FUNCTION_BLOCK FB_DO_IED_LD1_MMXU1_TotW EXTENDS FB_AcsiCommonDataClass
VAR_INPUT
	mag: FB_AcsiDATypeAnalogueValue := (fc:=ACSI_FC_MX, TrgOp:=ACSI_TrgOp_dchg OR ACSI_TrgOp_dupd, bLinkResult:=THIS^.AddDataToContainer(ipData:=mag));
	q: FB_AcsiDATypeQuality := (fc:=ACSI_FC_MX, TrgOp:=ACSI_TrgOp_qchg, bLinkResult:=THIS^.AddDataToContainer(ipData:=q));
	t: FB_AcsiDATypeTimeStamp := (fc:=ACSI_FC_MX, bLinkResult:=THIS^.AddDataToContainer(ipData:=t));
	units: FB_AcsiDATypeUnit := (fc:=ACSI_FC_CF, TrgOp:=ACSI_TrgOp_dchg, SIUnit:=(eValue:=E_AcsiSIUnit.Volt), multiplier:=(eValue:=E_AcsiMultiplier.Milli, bPresence:=TRUE), bLinkResult:=THIS^.AddDataToContainer(ipData:=units));
	db: FB_AcsiBATypeINT32U := (fc:=ACSI_FC_CF, TrgOp:=ACSI_TrgOp_dchg, bLinkResult:=THIS^.AddDataToContainer(ipData:=db));
	zeroDb: FB_AcsiBATypeINT32U := (fc:=ACSI_FC_CF, TrgOp:=ACSI_TrgOp_dchg, bLinkResult:=THIS^.AddDataToContainer(ipData:=zeroDb));
	sVC: FB_AcsiDATypeScaledValueConfig := (fc:=ACSI_FC_CF, TrgOp:=ACSI_TrgOp_dchg, bLinkResult:=THIS^.AddDataToContainer(ipData:=sVC));
	rangeC: FB_AcsiDATypeRangeConfig := (fc:=ACSI_FC_CF, TrgOp:=ACSI_TrgOp_dchg, hhLim:=(), hLim:=(), lLim:=(), llLim:=(), min_:=(), max_:=(), bLinkResult:=THIS^.AddDataToContainer(ipData:=rangeC));
	smpRate: FB_AcsiBATypeINT32U := (fc:=ACSI_FC_CF, TrgOp:=ACSI_TrgOp_dchg, bLinkResult:=THIS^.AddDataToContainer(ipData:=smpRate));
END_VAR
VAR
END_VAR

END_FUNCTION_BLOCK
